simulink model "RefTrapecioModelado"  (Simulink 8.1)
settings: Solver=ode4  StartTime=0.0  StopTime=tmax  FixedStep=1e-3  MaxStep=1e-3  MinStep=1e-3  RelTol=1e-3
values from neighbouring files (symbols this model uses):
  incp = 2    [RefTrapecioModeladoM.m]
  K0 = Km/p    (= 1.51515151515)    [RefTrapecioModeladoM.m]
  kInt = 2/(-t1+t2+t3)    (= 0.00571428571429)    [RefTrapecioModeladoM.m]    (also in RefTrapecioParam.m = 2/(-t1+t2+t3))
  Km = 100    [RefTrapecioModeladoM.m]    (also in RefTrapecioM.m)
  m1 = 0.15    [RefTrapecioModeladoM.m]    (also in RefTrapecioM.m; RefTrapecioParam.m)
  m2 = 0    [RefTrapecioModeladoM.m]    (also in RefTrapecioM.m = 0.075; RefTrapecioParam.m = 0.075)
  p = 66','Color','r')    [RefTrapecioModeladoM.m]    (also in RefTrapecioM.m = 66)
  t1 = 50    [RefTrapecioModeladoM.m]    (also in RefTrapecioParam.m)
  t2 = 200    [RefTrapecioModeladoM.m]    (also in RefTrapecioM.m; RefTrapecioParam.m)
libraries: simulink x5

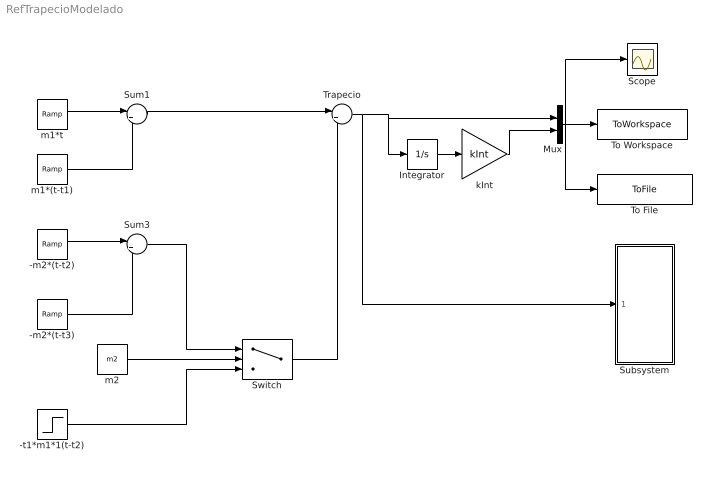
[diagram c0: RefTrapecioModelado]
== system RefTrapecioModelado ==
  -m2*(t-t2) : simulink/Sources/Ramp  slope=-m2  start=t2  X0=0
  -m2*(t-t3) : simulink/Sources/Ramp  slope=-m2  start=t3  X0=0
  -t1*m1*1(t-t2) : Step  Time=t2  After=-t1*m1  SampleTime=0
  Integrator : Integrator
  Mux : Mux  Inputs=2
  Scope : Scope
  Subsystem : Subsystem
  Sum1 : Sum  Inputs=|+-
  Sum3 : Sum  Inputs=|+-
  Switch : Switch  Criteria=u2 > Threshold  OutDataTypeStr=double  SampleTime=0
  To File : ToFile  Filename=TrapecioInt.mat
  To Workspace : ToWorkspace  VariableName=TrapecioInt  SampleTime=-1
  Trapecio : Sum  Inputs=|++
  kInt : Gain  Gain=kInt
  m1*(t-t1) : simulink/Sources/Ramp  slope=m1  start=t1  X0=0
  m1*t : simulink/Sources/Ramp  slope=m1  start=0  X0=0
  m2 : Constant  Value=m2
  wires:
  -m2*(t-t2)/1 -> Sum3/1
  m1*(t-t1)/1 -> Sum1/2
  Sum1/1 -> Trapecio/1
  m1*t/1 -> Sum1/1
  Trapecio/1 -> Subsystem/1(u(t)), Integrator/1, Mux/1
  Mux/1 -> Scope/1, To Workspace/1, To File/1
  Integrator/1 -> kInt/1
  kInt/1 -> Mux/2
  m2/1 -> Switch/2
  -m2*(t-t3)/1 -> Sum3/2
  Sum3/1 -> Switch/1
  Switch/1 -> Trapecio/2
  -t1*m1*1(t-t2)/1 -> Switch/3

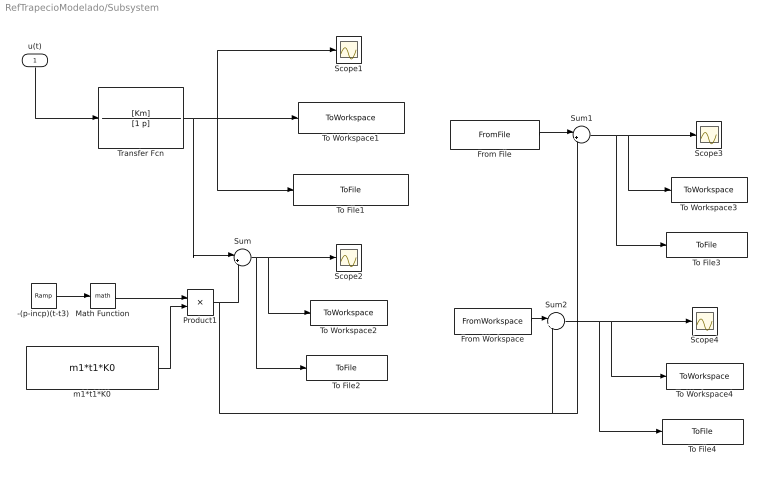
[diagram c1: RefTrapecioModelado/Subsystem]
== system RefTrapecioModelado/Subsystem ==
  u(t) : Inport
  -(p-incp)(t-t3) : simulink/Sources/Ramp  slope=-p+incp  start=t3  X0=0
  From Workspace : FromWorkspace  VariableName=DatosArray  SampleTime=0
  From File : FromFile  FileName=DatosSistema.mat  SampleTime=0
  Math Function : Math  OutputSignalType=real
  Product1 : Product
  Scope{1..4} (4 alike) : Scope
  Sum : Sum  Inputs=|+-  SampleTime=0
  Sum1 : Sum  Inputs=|+-  SampleTime=0
  Sum2 : Sum  Inputs=|+-  SampleTime=0
  To File1 : ToFile  Filename=TrapecioOrdenUno.mat
  To File2 : ToFile  Filename=Error.mat
  To File3 : ToFile  Filename=ErrorB.mat
  To File4 : ToFile  Filename=ErrorB1.mat
  To Workspace1 : ToWorkspace  VariableName=TrapecioOrdenUno  SampleTime=-1
  To Workspace2 : ToWorkspace  VariableName=Error  SampleTime=-1
  To Workspace3 : ToWorkspace  VariableName=ErrorB  SampleTime=-1
  To Workspace4 : ToWorkspace  VariableName=ErrorB1  SampleTime=-1
  Transfer Fcn : TransferFcn  Numerator=[Km]  Denominator=[1 p]
  m1*t1*K0 : Constant  Value=m1*t1*K0
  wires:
  -(p-incp)(t-t3)/1 -> Math Function/1
  Sum/1 -> To File2/1, To Workspace2/1, Scope2/1
  u(t)/1 -> Transfer Fcn/1
  m1*t1*K0/1 -> Product1/2
  Math Function/1 -> Product1/1
  Transfer Fcn/1 -> Sum/1, To File1/1, To Workspace1/1, Scope1/1
  Sum1/1 -> To File3/1, To Workspace3/1, Scope3/1
  From File/1 -> Sum1/1
  Product1/1 -> Sum/2, Sum1/2, Sum2/2
  Sum2/1 -> To File4/1, To Workspace4/1, Scope4/1
  From Workspace/1 -> Sum2/1
